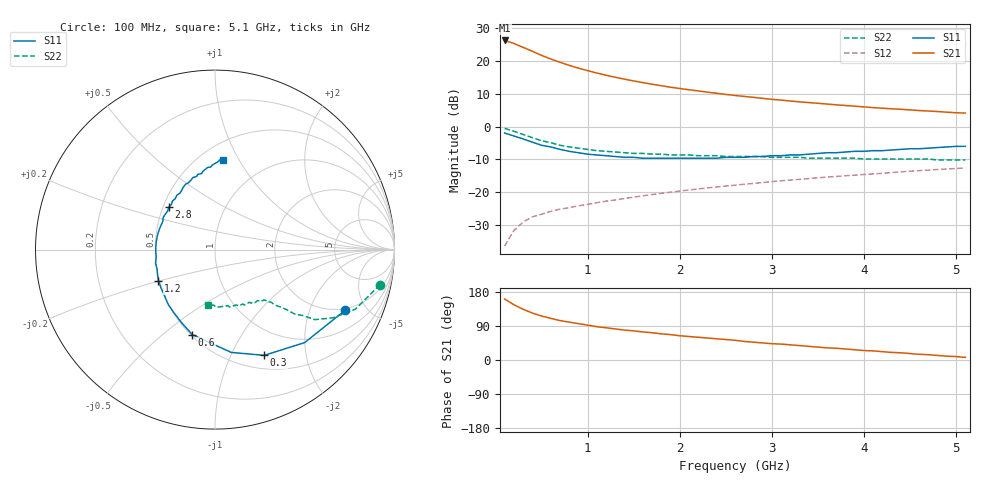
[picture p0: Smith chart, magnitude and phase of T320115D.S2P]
!AT-32011
!S PARAMETERS at Vce=5  V  Ic=7.5mA.  LAST UPDATED 01-05-95
# ghz s ma r 50
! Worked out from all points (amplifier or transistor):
!   51 points, 100 MHz to 5.1 GHz, reference 50 ohm
!   highest |S21| = 26.3 dB at 100 MHz (marker M1)
!   |S21| within 3 dB of that: start of sweep to 375.6 MHz
!   unconditionally stable (mu >= 1): 1.625 GHz to 4.936 GHz
!   at 900 MHz: K = 0.77, MSG = 21.0 dB, |S12| = -24.2 dB
!   at 2.6 GHz: K = 1.09, MAG = 11.9 dB, |S12| = -17.9 dB
!   at 5.1 GHz: K = 0.99, MSG = 8.4 dB, |S12| = -12.6 dB
!   S11 on the Smith chart (normalised r, x): 100 MHz: 1.90, -3.56; 300 MHz: 0.66, -1.35; 600 MHz: 0.51, -0.63; 1.2 GHz: 0.49, -0.20; 2.8 GHz: 0.54, +0.29; 5.1 GHz: 0.64, +0.86
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0.1  0.8 -25.0  20.65 161.0  0.015 77.0  0.94 -12.0
0.2  0.72 -46.0  18.57 146.0  0.026 68.0  0.85 -23.0
0.3  0.65 -65.0  16.24 134.0  0.035 61.0  0.76 -30.0
0.4  0.58 -81.0  14.13 124.0  0.042 57.0  0.68 -35.0
0.5  0.52 -93.0  12.24 116.0  0.046 54.0  0.61 -37.0
0.6  0.49 -105.0  10.78 110.0  0.051 53.0  0.57 -39.0
0.7  0.45 -114.0  9.6 104.0  0.055 52.0  0.52 -40.0
0.8  0.42 -123.0  8.62 100.0  0.058 52.0  0.49 -41.0
0.9  0.4 -131.0  7.82 96.0  0.062 52.0  0.47 -42.0
1  0.38 -138.0  7.15 92.0  0.065 52.0  0.45 -43.0
1.1  0.37 -144.0  6.58 88.0  0.069 52.0  0.43 -43.0
1.2  0.36 -151.0  6.09 85.0  0.073 52.0  0.42 -44.0
1.4  0.34 -162.0  5.31 79.0  0.08 52.0  0.4 -45.0
1.6  0.33 -173.0  4.7 74.0  0.088 52.0  0.39 -47.0
1.8  0.33 178.0  4.21 69.0  0.096 52.0  0.38 -49.0
2.1  0.33 164.0  3.65 62.0  0.108 51.0  0.37 -53.0
2.6  0.34 144.0  2.99 52.0  0.128 49.0  0.35 -58.0
2.8  0.35 137.0  2.8 47.0  0.136 48.0  0.35 -61.0
3  0.36 131.0  2.61 43.0  0.145 47.0  0.34 -63.0
3.5  0.39 117.0  2.27 34.0  0.166 45.0  0.33 -70.0
4.3  0.44 99.0  1.87 20.0  0.199 40.0  0.32 -81.0
5.1  0.5 85.0  1.61 7.0  0.235 33.0  0.31 -97.0
